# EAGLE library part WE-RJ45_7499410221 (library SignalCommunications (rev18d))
WE-RJ45 LAN Transformer Order Code 7499410221 Design THT xBase-T 10/100 Base-T Ports 1x1 Application Standard Tab Position Vertical LED (Left-Right) GREEN-GREEN EMI Fingers No Details see: http://katalog.we-online.de/en/pbs/WE-LAN-RJ45 Created by Yingchun Shan 2016 (C) Wurth Elektronik
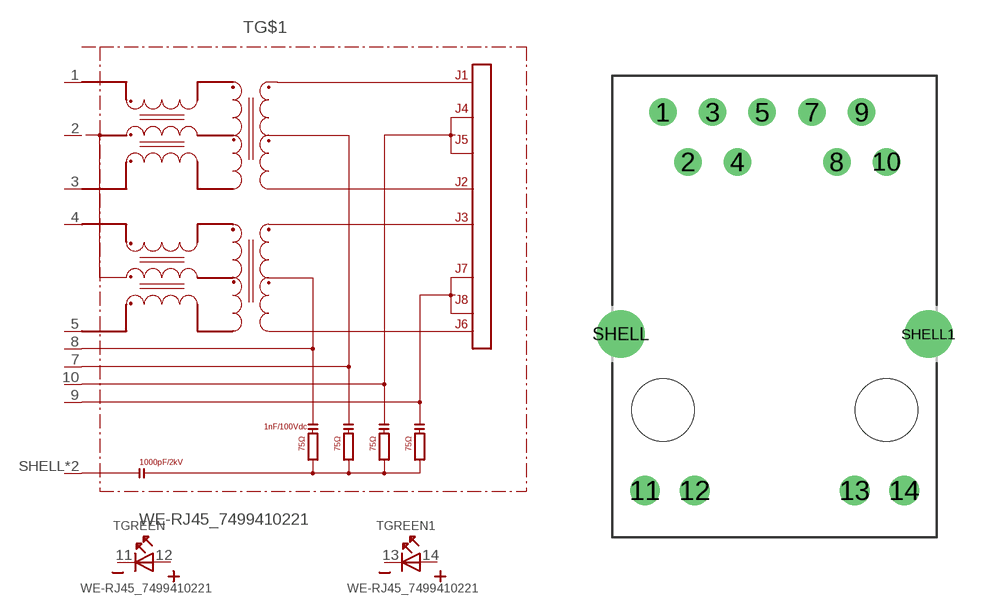
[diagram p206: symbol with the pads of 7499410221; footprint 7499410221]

Designator prefix T; gates G$1=7499410221 GREEN=LED_2PIN GREEN1=LED_2PIN

## WE-RJ45_7499410221  [7499410221]
1  G$1:P1
2  G$1:P2
3  G$1:P3
4  G$1:P4
5  G$1:P5
7  G$1:P7
8  G$1:P8
9  G$1:P9
10  G$1:P10
11  GREEN:K  pas
12  GREEN:A  pas
13  GREEN1:K  pas
14  GREEN1:A  pas
SHELL  G$1:SHIELD
SHELL1  G$1:SHIELD

## Footprint 7499410221 (pad centres in mm)
drill 0.9: 1 -5.72,15.24; 2 -4.44,12.7; 3 -3.18,15.24; 4 -1.9,12.7; 5 -0.64,15.24; 7 1.9,15.24; 8 3.18,12.7; 9 4.44,15.24; 10 5.72,12.7
drill 1.02: 11 -6.635,-4.11; 12 -4.095,-4.11; 13 4.095,-4.11; 14 6.635,-4.11
drill 1.63: SHELL -7.875,3.89; SHELL1 7.875,3.89
hole 3.2 at -5.715,0
hole 3.2 at 5.715,0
